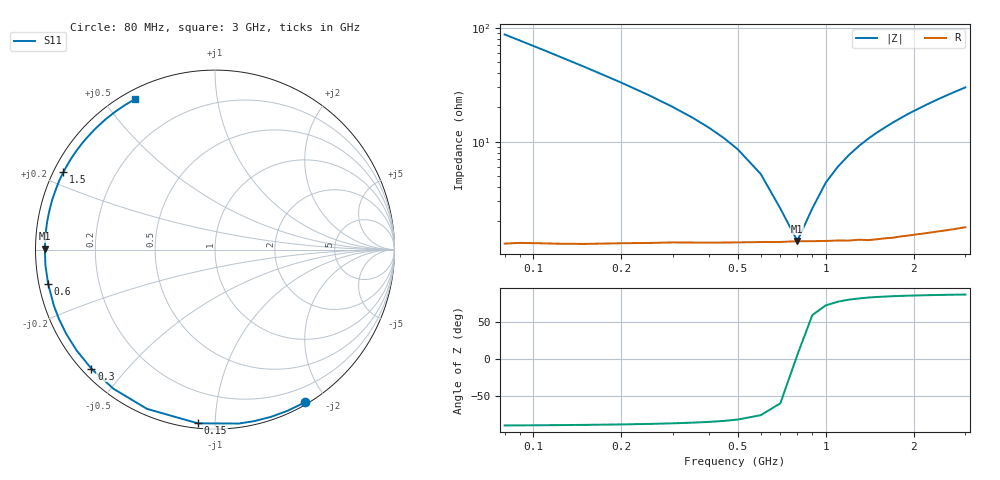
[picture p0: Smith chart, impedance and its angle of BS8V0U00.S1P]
! SIEMENS Small Signal Semiconductors
! BB640
! Si Tuning Diode in SOD323
! VR = 8 V
! S-Parameters:  July  1993
# GHz  S  MA  R  50
!  f  S11
! GHz  MAG  ANG
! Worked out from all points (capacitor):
!   33 points, 80 MHz to 3 GHz, reference 50 ohm
!   read as one part to ground: C = 22.6 pF near 80 MHz
!   lowest |Z| = 1.34 ohm at 800 MHz (marker M1)
!   series resonance near 794.4 MHz, so ESL is about 1.8 nH
!   S11 on the Smith chart (normalised r, x): 80 MHz: 0.03, -1.75; 150 MHz: 0.03, -0.91; 300 MHz: 0.03, -0.40; 600 MHz: 0.03, -0.10; 1.5 GHz: 0.03, +0.24; 3 GHz: 0.04, +0.60
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0.08  0.9875 -59.6
0.09  0.9849 -65.7
0.1  0.9826 -71.5
0.11  0.9804 -76.9
0.12  0.9783 -82.1
0.15  0.9726 -95.6
0.2  0.9649 -113.1
0.25  0.9598 -126.1
0.3  0.9561 -136.1
0.35  0.954 -144.0
0.4  0.9526 -150.5
0.45  0.9514 -156.0
0.5  0.9505 -160.7
0.6  0.9493 -168.5
0.7  0.9488 -174.9
0.8  0.9479 179.7
0.9  0.948 174.9
1  0.948 170.5
1.2  0.9484 162.9
1.4  0.949 156.1
1.5  0.9487 153.0
1.6  0.9484 150.1
1.8  0.948 144.5
2  0.9478 139.3
2.2  0.9479 134.5
2.4  0.948 130.0
2.8  0.9487 121.9
3  0.9491 118.2
